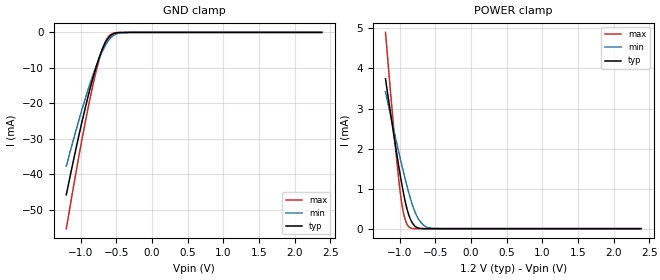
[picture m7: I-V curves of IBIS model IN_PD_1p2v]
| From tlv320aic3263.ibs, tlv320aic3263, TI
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|   IN_PD_1p2v
[Model]   IN_PD_1p2v
Model_type   Input
Vinl = 1.08
Vinh = 0.12
|   typ   min   max
C_comp   1.100pF   1.086pF   1.128pF
[Voltage Range]   1.2   1.1   1.3
[Temperature Range]   27   125   -40
[Power Clamp Reference]   1.2   1.1   1.3
[GND Clamp Reference]   -0   -0   -0
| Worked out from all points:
|   GND clamp passes 1 mA (typ) near -0.58 V on its own axis
|   POWER clamp passes 1 mA (typ) near -0.96 V on its own axis
[GND Clamp]
|   Voltage   I(typ)   I(min)   I(max)
-1.2V     -45.78mA   -37.73mA   -55.33mA
-1.11V    -37.06mA   -30.96mA   -44.72mA
-984mV    -25.55mA   -22.02mA   -30.58mA
-894mV    -18.01mA   -16.12mA   -21.24mA
-822mV    -12.53mA   -11.79mA   -14.42mA
-750mV    -7.751mA   -7.917mA   -8.473mA
-696mV    -4.78mA    -5.405mA   -4.842mA
-642mV    -2.508mA   -3.332mA   -2.212mA
-588mV    -1.053mA   -1.79mA    -741.2uA
-480mV    -90.6uA    -311.8uA   -33.7uA
-300mV    -390.3nA   -5.742uA   -92.72nA
2.382V    0A         0A         0A
[POWER Clamp]
|   Voltage   I(typ)   I(min)   I(max)
-1.2V     3.742mA    3.419mA    4.901mA
-1.074V   2.231mA    2.387mA    2.298mA
-1.002V   1.428mA    1.82mA     1.03mA
-966mV    1.06mA     1.547mA    562.4uA
-930mV    731.2uA    1.283mA    261.5uA
-894mV    461.8uA    1.032mA    95.66uA
-858mV    267.1uA    798.5uA    24.89uA
-804mV    94.1uA     498uA      2.317uA
-732mV    11.85uA    224.2uA    130.7nA
-660mV    977.7nA    77.56uA    51.68nA
-534mV    32.77nA    4.319uA    48.77nA
2.382V    0A         0A         0A
